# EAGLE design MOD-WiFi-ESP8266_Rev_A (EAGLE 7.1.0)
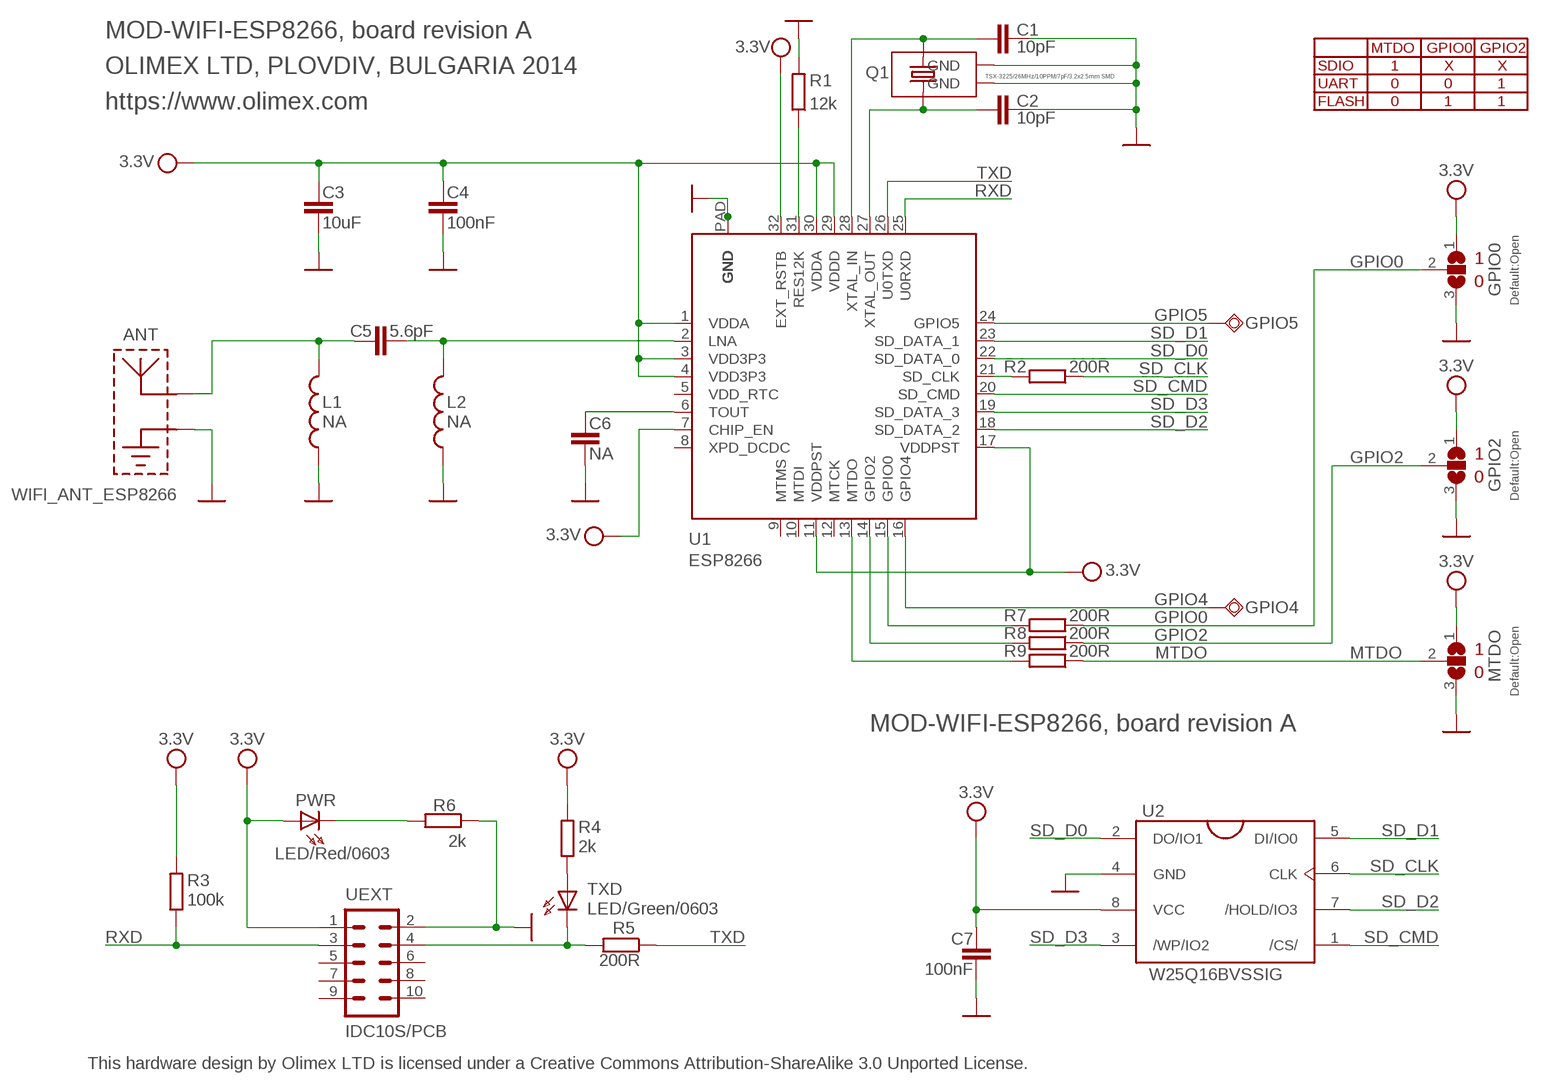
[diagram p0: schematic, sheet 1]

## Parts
ANT  WIFI_ANT_ESP8266  [ESP8266_ANT]
C1  10pF  C-EUC0402_TI  [C0402_TI]
C2  10pF  C-EUC0402_TI  [C0402_TI]
C3  10uF  C-EUC0603_DWS  [C0603_DWS]
C4  100nF  C-EUC0402_TI  [C0402_TI]
C5  5.6pF  C-EUC0402_TI  [C0402_TI]
C6  NA  C-EUC0402_TI  [C0402_TI]
C7  100nF  C-EUC0402_TI  [C0402_TI]
GPIO0  Default:Open  SJ2W4  [SJ_2_SMALLER]
GPIO2  Default:Open  SJ2W4  [SJ_2_SMALLER]
GPIO4  TESTPAD32/56  [TESTPAD32/56]
GPIO5  TESTPAD32/56  [TESTPAD32/56]
L1  NA  L-USL0402_TI  [L0402_TI]
L2  NA  L-USL0402_TI  [L0402_TI]
MTDO  Default:Open  SJ2W4  [SJ_2_SMALLER]
PWR  LED/Red/0603  LED0603DWS  [LED-0603]
Q1  TSX-3225/26MHz/10PPM/7pF/3.2x2.5mm SMD  SMALL_SMD_CRYSTAL_1  [NX3225SA]
R1  12k  R-EU_R0402_TI  [R0402_TI]
R2  200R  R-EU_R0402_TI  [R0402_TI]
R3  100k  R-EU_R0402_TI  [R0402_TI]
R4  2k  R-EU_R0402_TI  [R0402_TI]
R5  200R  R-EU_R0402_TI  [R0402_TI]
R6  2k  R-EU_R0402_TI  [R0402_TI]
R7  200R  R-EU_R0402_TI  [R0402_TI]
R8  200R  R-EU_R0402_TI  [R0402_TI]
R9  200R  R-EU_R0402_TI  [R0402_TI]
TXD  LED/Green/0603  LED0603DWS_L  [LED-0603_L]
U1  ESP8266  [QFN32_PAD]
U2  W25Q16BVSSIG  [SO8_ATMEL_FLASH]
UEXT  IDC10S/PCB  ML10SMD_1  [ML10L_PADS_FEMAIL]

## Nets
GND: ANT.GND C1.1 C2.1 C3.2 C4.2 C6.2 C7.2 GPIO0.3 GPIO2.3 L1.1 L2.1 MTDO.3 Q1.NC_1(GND) Q1.NC_2(GND) R1.2 R6.1 U1.P$1(GND) U1.P$2(GND) U1.P$3(GND) U1.P$4(GND) U1.P$5(GND) U1.P$6(GND) U1.P$7(GND) U1.P$8(GND) U1.P$9(GND) U1.PAD(GND) U2.4(GND) UEXT.2
GPIO0: GPIO0.2 R7.1
GPIO2: GPIO2.2 R8.1
GPIO4: GPIO4.P$1(PP) U1.16(GPIO4)
GPIO5: GPIO5.P$1(PP) U1.24(GPIO5)
MTDO: MTDO.2 R9.1
N$1: R5.2 TXD.C UEXT.4
N$2: R4.1 TXD.A
N$3: PWR.C R6.2
N$4: R7.2 U1.15(GPIO0)
N$5: R8.2 U1.14(GPIO2)
N$6: R9.2 U1.13(MTDO)
N$12: C5.2 L2.2 U1.2(LNA)
N$14: ANT.ANT C5.1 L1.2
N$18: C6.1 U1.6(TOUT)
N$21: C2.2 Q1.2 U1.27(XTAL_OUT)
N$22: R1.1 U1.31(RES12K)
N$23: C1.2 Q1.1 U1.28(XTAL_IN)
N$27: R2.2 U1.21(SD_CLK)
RXD: R3.1 U1.25(U0RXD) UEXT.3
SD_CLK: R2.1 U2.6(CLK)
SD_CMD: U1.20(SD_CMD) U2.1(/CS/)
SD_D0: U1.22(SD_DATA_0) U2.2(DO/IO1)
SD_D1: U1.23(SD_DATA_1) U2.5(DI/IO0)
SD_D2: U1.18(SD_DATA_2) U2.7(/HOLD/IO3)
SD_D3: U1.19(SD_DATA_3) U2.3(/WP/IO2)
TXD: R5.1 U1.26(U0TXD)
VCC: C3.1 C4.1 C7.1 GPIO0.1 GPIO2.1 MTDO.1 PWR.A R3.2 R4.2 U1.1(VDDA) U1.3(VDD3P3) U1.4(VDD3P3) U1.7(CHIP_EN) U1.11(VDDPST) U1.17(VDDPST) U1.29(VDDD) U1.30(VDDA) U1.32(EXT_RSTB) U2.8(VCC) UEXT.1 ; supply symbol labelled 3.3V
Unconnected: U1.5(VDD_RTC) U1.8(XPD_DCDC) U1.9(MTMS) U1.10(MTDI) U1.12(MTCK) UEXT.5 UEXT.6 UEXT.7 UEXT.8 UEXT.9 UEXT.10

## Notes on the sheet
- MOD-WIFI-ESP8266, board revision A
- MTDO | GPIO0 | GPIO2
- OLIMEX LTD, PLOVDIV, BULGARIA 2014 | SDIO | 1 | X | X
- UART | 0 | 0 | 1
- https://www.olimex.com | FLASH | 0 | 1 | 1
- 1
- 0
- 1
- 0
- 1
- 0
- MOD-WIFI-ESP8266, board revision A
- This hardware design by Olimex LTD is licensed under a Creative Commons Attribution-ShareAlike 3.0 Unported License.

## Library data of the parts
ANT = OLIMEX_ANT:WIFI_ANT_ESP8266
C1-C7 = rcl:C-EU: CAPACITOR, European symbol
GPIO0 GPIO2 MTDO = jumper:SJ2W: SMD solder JUMPER
GPIO4 GPIO5 = gogo:TESTPAD: drill 40mils, diameter 70mils
L1 L2 = rcl:L-US: INDUCTOR, American symbol
PWR TXD = DOUBLE-SIDE:LED
Q1 = OLIMEX_DISCRET:SMALL_SMD_CRYSTAL
R1-R9 = rcl:R-EU_: RESISTOR, European symbol
U1 = OLIMEX_IC:ESP8266
U2 = OLIMEX_IC:W25Q16BVSSIG
UEXT = con-harting-ml:ML10: HARTING

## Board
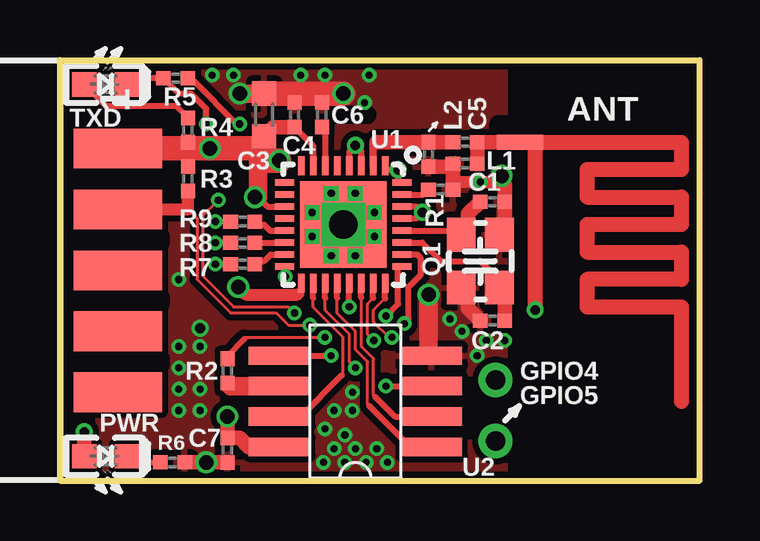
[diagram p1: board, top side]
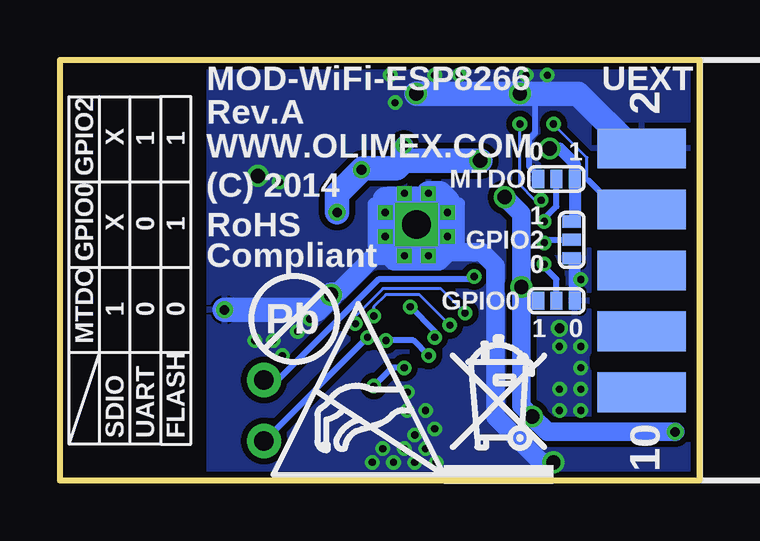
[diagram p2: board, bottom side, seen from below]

Size 26.67 x 17.53 mm. Coordinates in mm from the lower left corner, seen from the top.
Outline: 26.67,0 26.67,17.53 0,17.53 0,0 26.67,0
Copper layers (1+16): Top 0.035mm / dielectric 1.5mm / Bottom 0.035mm
Design rules "default": minimum track width 5mil, minimum drill 0.3mm, track to track 5mil, track to pad 5mil, pad to pad 5mil, via to via 5mil, smd to smd 1mil, copper to edge 5mil, drill to drill 8mil, minimum pad ring 6mil, minimum via ring 6mil, stop-mask expansion 2mil, vias tented up to drill 25mil, thermal gap 10mil
tRestrict: 6 lines
bRestrict: 7 lines

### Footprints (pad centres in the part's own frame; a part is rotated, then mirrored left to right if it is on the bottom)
ESP8266_ANT = smd 0.635 x 1.905: ANT -5.334,-3.302 | drill 0.4 pad 0.635: GND 1.651,-2.667
C0402_TI = smd 0.61 x 0.584: 1 -0.508,0; 2 0.508,0
C0603_DWS = smd 1.016 x 1.016: 1 -0.889,0; 2 0.889,0
SJ_2_SMALLER = smd 0.508 x 0.762: 1 -0.762,0; 2 0,0; 3 0.762,0
TESTPAD32/56 = drill 0.813 pad 1.422: P$1 0,0
L0402_TI = smd 0.61 x 0.584: 1 -0.508,0; 2 0.508,0
LED-0603 = smd 1.016 x 1.016: A 0.889,0; C -0.889,0
NX3225SA = smd 1.4 x 1.2: 1 -1.1,-0.8; 2 1.1,0.8; NC_1 1.1,-0.8; NC_2 -1.1,0.8
R0402_TI = smd 0.61 x 0.584: 1 -0.508,0; 2 0.508,0
LED-0603_L = smd 1.016 x 1.016: A 0.889,0; C -0.889,0
QFN32_PAD = smd 0.8 x 0.28: 1 -2.45,1.75; 2 -2.45,1.25; 3 -2.45,0.75; 4 -2.45,0.25; 5 -2.45,-0.25; 6 -2.45,-0.75; 7 -2.45,-1.25; 8 -2.45,-1.75; 17 2.45,-1.75; 18 2.45,-1.25; 19 2.45,-0.75; 20 2.45,-0.25; 21 2.45,0.25; 22 2.45,0.75; 23 2.45,1.25; 24 2.45,1.75 | smd 0.28 x 0.8: 9 -1.75,-2.45; 10 -1.25,-2.45; 11 -0.75,-2.45; 12 -0.25,-2.45; 13 0.25,-2.45; 14 0.75,-2.45; 15 1.25,-2.45; 16 1.75,-2.45; 25 1.75,2.45; 26 1.25,2.45; 27 0.75,2.45; 28 0.25,2.45; 29 -0.25,2.45; 30 -0.75,2.45; 31 -1.25,2.45; 32 -1.75,2.45 | drill 1.2 pad 1.422 square: P$1 0,0 | drill 0.3 pad 0.4 square: P$2 0.5,1.3; P$3 -0.5,1.3; P$4 -1.3,0.5; P$5 -1.3,-0.5; P$6 -0.5,-1.3; P$7 0.5,-1.3; P$8 1.3,-0.5; P$9 1.3,0.5 | smd 3.6 x 3.6: PAD 0,0
SO8_ATMEL_FLASH = smd 0.762 x 2.54: 1 -1.905,-3.175; 2 -0.635,-3.175; 3 0.635,-3.175; 4 1.905,-3.175; 5 1.905,3.175; 6 0.635,3.175; 7 -0.635,3.175; 8 -1.905,3.175
ML10L_PADS_FEMAIL = smd 1.651 x 3.683 bottom: 1 -5.08,-3.429; 3 -2.54,-3.429; 5 0,-3.429; 7 2.54,-3.429; 9 5.08,-3.429 | smd 1.651 x 3.683: 2 -5.08,-3.429; 4 -2.54,-3.429; 6 0,-3.429; 8 2.54,-3.429; 10 5.08,-3.429

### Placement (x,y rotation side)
ANT  22.48,8.76 270 top
C1  18.03,11.62 180 top
C2  18.03,6.67 0 top
C3  8.51,15.24 90 top
C4  9.78,15.24 90 top
C5  16.89,14.1 180 top
C6  10.92,15.24 90 top
C7  6.99,1.27 270 top
GPIO0  5.97,7.49 0 bottom
GPIO2  5.33,10.03 270 bottom
GPIO4  18.16,4.19 0 top
GPIO5  18.16,1.65 0 top
L1  16.89,13.21 0 top
L2  15.37,13.59 90 top
MTDO  5.97,12.57 180 bottom
PWR  1.91,1.02 180 top
Q1  17.53,9.14 270 top
R1  15.88,12.13 0 top
R2  6.99,4.57 90 top
R3  5.33,12.57 90 top
R4  5.33,14.61 270 top
R5  4.83,16.76 180 top
R6  4.7,0.76 180 top
R7  7.62,9.02 0 top
R8  7.62,9.91 0 top
R9  7.62,10.79 0 top
TXD  1.91,16.51 180 top
U1  11.81,10.67 270 top
U2  12.32,3.3 90 top
U$4  [ESD_SYMBOL]  17.78,0.25 0 bottom
U$6  [PB_SMALL]  16.89,6.73 180 bottom
U$7  [RECYCLE_BIN1/8]  10.67,-0.13 0 bottom
UEXT  -1.02,8.76 270 bottom

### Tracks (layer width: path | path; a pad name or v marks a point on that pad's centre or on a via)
GND  (via drill 0.3, 0.4, 0.6)
  Top 0.254: 17.02,8.04 Q1.NC_1
  Top 0.508: 16.38,12.45 18.41,12.45 v18.41,12.7
  Top 0.61: 16.38,13.08 L2.1 | R1.2 16.38,12.45 16.38,13.08 | 16.38,13.08 L1.1 | Q1.NC_2 18.54,10.46 C1.1 18.54,12.32 18.41,12.45 | C2.1 17.02,7.18 17.02,8.04 | R6.1 v6.1,0.76 C7.2 | 9.78,16.13 C4.2 | 10.92,16.13 C6.2
  Top 0.762: v15.37,7.75 15.37,5.21 U2.4 | v7.49,16.13 C3.2
  Top 1.016: C3.2 9.78,16.13 10.92,16.13 v11.81,16.13
  Bottom 0.254: MTDO.3 6.73,12.7 7.11,13.08 7.11,14.22 6.86,14.48 6.86,16.13
  Bottom 0.508: 13.11,11.72 12.95,11.87 | U1.P$5 11.31,11.87 | 12.31,11.87 U1.P$4 | 10.03,11.56 10.03,9.78 10.79,9.02 12.83,9.02 13.59,9.78 13.59,11.56 13.11,11.56 | GPIO0.3 5.21,9.27 GPIO2.3
  Bottom 0.762: v6.1,0.76 6.6,0.76 8.51,2.67 8.51,8.95 9.08,9.53 10.67,9.53 | 12.95,11.87 12.31,11.87 11.31,11.87 | 12.8,9.37 13.56,9.37 15.05,7.87 15.24,7.87 v15.37,7.75
  Bottom 1.016: UEXT.2 2.79,13.84 5.08,16.13 6.86,16.13 v7.49,16.13 v11.81,16.13 | 13.11,11.72 13.11,11.56 U1.P$3 U1.P$2 13.11,9.68 12.8,9.37 U1.P$9 U1.P$8 10.82,9.37 10.67,9.53 10.51,9.68 U1.P$7 10.51,10.67 | U1.P$5 10.82,11.97 10.51,11.65 U1.P$6 10.51,10.67 | 10.51,10.67 U1.P$1 | v15.37,7.75 16,7.11 ANT.GND
  other vias: 5.84,6.35 5.84,5.59 4.95,5.59 4.95,4.7 4.95,3.81 5.84,3.81 4.95,2.92 11.43,2.92 11.05,2.16 11.87,0.76 10.99,0.76 13.65,0.76 13.21,1.33 12.76,0.76 12.32,1.33 11.43,1.33 11.87,1.91 12.19,2.92 12.19,3.68 16.26,6.73 16.76,6.22 12.7,15.75 17.53,12.45 4.95,8.38 5.84,2.92 12.89,16.89 17.4,5.21 18.54,5.84 17.78,5.84 10.03,16.89 11.05,16.89 7.24,16.89 6.35,16.89
  pour Top (isolate 0.254): -2.54,-2.54 -2.54,20.07 29.21,20.07 29.21,-2.54
  pour Bottom (isolate 0.254): -5.08,-5.08 -5.08,22.61 31.88,22.61 31.88,-5.08
GPIO0  (via drill 0.3)
  Top 0.254: v6.48,9.02 R7.1
  Bottom 0.254: v6.48,9.02 6.48,8.89 5.97,8.38 GPIO0.2
GPIO2  (via drill 0.3)
  Top 0.254: R8.1 v6.48,9.91
  Bottom 0.254: v6.48,9.91 6.35,10.03 GPIO2.2
GPIO4  (via drill 0.3)
  Top 0.254: U1.16 9.4,8.92 v9.4,8.51
  Bottom 0.254: v9.4,8.51 9.53,8.38 13.4,8.38 17.59,4.19 GPIO4.P$1
GPIO5  (via drill 0.3)
  Top 0.127: 13.56,7.59 13.08,7.11 13.08,6.6 13.72,5.97 v13.84,5.97
  Top 0.254: 13.56,7.59 U1.24
  Bottom 0.254: GPIO5.P$1 v13.84,5.97
MTDO  (via drill 0.3)
  Top 0.254: R9.1 v6.48,10.79
  Bottom 0.254: v6.48,10.79 6.48,10.92 5.97,11.43 MTDO.2
N$1  (via drill 0.3)
  Top 0.254: TXD.C 3.05,16.76 R5.2 4.95,16.13 5.46,16.13 6.1,15.49 v6.1,14.86
  Bottom 0.127: UEXT.4 3.43,11.3 | 4.64,12.51 4.7,12.57 4.7,13.46 v6.1,14.86
  Bottom 0.254: 3.43,11.3 4.64,12.51
N$2
  Top 0.254: TXD.A 1.91,15.62 4.83,15.62 R4.1
N$3
  Top 0.254: PWR.C 3.05,0.76 R6.2
N$4
  Top 0.254: R7.2 8.26,9.14 8.51,9.14 8.78,9.42 U1.15
N$5
  Top 0.254: R8.2 U1.14
N$6
  Top 0.254: R9.2 8.26,10.67 8.51,10.67 8.76,10.42 U1.13
N$12
  Top 0.305: U1.2 13.06,13.95 13.21,14.1
  Top 0.61: C5.2 L2.2 13.21,14.1
N$14
  Top 0.61: L1.2 C5.1 ANT.ANT
N$18
  Top 0.254: C6.1 11.06,14.59 U1.6
N$21
  Top 0.254: U1.27 15.1,9.92 15.88,9.14 17.53,9.14 18.33,8.34 Q1.2
  Top 0.61: C2.2 18.54,7.83 Q1.2
N$22
  Top 0.254: U1.31 15.16,11.92 R1.1
N$23
  Top 0.254: 17.02,10.24 Q1.1 | U1.28 17.02,10.42
  Top 0.61: 17.02,10.24 17.02,10.42 17.02,11.11 C1.2
N$27  (via drill 0.3)
  Top 0.127: v12.06,7.24 | R2.2 6.99,5.21 | 7.68,5.91 7.75,5.97 v11.05,5.97
  Top 0.254: v12.06,7.24 U1.21 | 6.99,5.21 7.68,5.91
  Bottom 0.254: v11.05,5.97 11.05,6.22 v12.06,7.24
RXD  (via drill 0.3)
  Top 0.127: 5.33,11.3 5.71,10.92 5.71,8.38 7.11,6.99 9.02,6.99 9.53,6.48 v10.41,6.48
  Top 0.254: v13.59,6.86 14.1,7.37 14.1,8.38 14.1,8.92 U1.25
  Top 0.508: UEXT.3 5.33,11.3 R3.1
  Bottom 0.127: v10.41,6.48 11.68,7.75 13.08,7.75 13.59,7.24 v13.59,6.86
SD_CLK
  Top 0.61: R2.1 7.11,3.94
  Top 0.762: 7.11,3.94 U2.6
SD_CMD
  Top 0.127: 12.89,3.11 12.83,3.17 12.83,4.95 12.32,5.46 12.32,6.22 11.56,6.98 11.56,7.62
  Top 0.254: 11.56,7.62 U1.20 | U2.1 14.61,1.4 12.89,3.11
SD_D0
  Top 0.127: 12.56,7.63 12.57,7.62 12.57,5.59 13.08,5.08 13.08,3.56 13.14,3.49
  Top 0.254: 12.56,7.63 U1.22 | 13.14,3.49 13.97,2.67 U2.2
SD_D1  (via drill 0.3)
  Top 0.127: v13.08,5.84 12.83,6.1 12.83,7.37 13.06,7.6
  Top 0.254: 13.06,7.6 U1.23 | U2.5 v11.3,5.21
  Bottom 0.254: v11.3,5.21 11.94,5.84 v13.08,5.84
SD_D2
  Top 0.127: 11.75,4.38 11.81,4.45 11.81,5.97 10.56,7.22 10.56,7.6 | U2.7 10.03,2.67
  Top 0.254: 10.56,7.6 U1.18 | 10.03,2.67 11.75,4.38
SD_D3  (via drill 0.3)
  Top 0.127: v12.32,4.7 12.06,4.95 12.06,6.1 11.06,7.1 11.06,7.61
  Top 0.254: 11.06,7.61 U1.19 | v13.59,3.94 U2.3
  Bottom 0.254: v12.32,4.7 12.83,4.7 v13.59,3.94
TXD  (via drill 0.3)
  Top 0.127: v6.6,11.68 5.97,11.05 5.97,8.51 7.24,7.24 9.53,7.24 v9.78,6.99
  Top 0.254: U1.26 14.9,9.42 15.05,9.27 15.05,8.57 14.54,8.06 14.54,6.73 v14.35,6.54 | v7.49,14.86 7.37,14.86 5.59,16.64 5.21,16.64 R5.1
  Bottom 0.127: v6.6,11.68 6.86,11.68 7.49,12.32 v7.49,14.86 | v14.35,6.54 14.35,6.86 13.21,8 10.79,8 v9.78,6.99
VCC  (via drill 0.4, 0.6)
  Top 0.254: C4.1 10.56,13.95 U1.7 | U1.4 12.06,13.71 v12.32,13.97 12.56,13.73 U1.3 | U1.1 13.56,12.95 v14.1,12.95 14.1,12.42 U1.32 | U1.30 14.87,11.42 v15.11,11.18 14.86,10.92 U1.29 | 9.91,7.75 10.06,7.75 U1.17 | 8.26,11.81 8.65,11.42 U1.11
  Top 0.508: v7.43,8.06 7.75,7.75 9.91,7.75
  Top 0.61: PWR.A v1.02,2.03 | v6.99,2.67 C7.1 7.49,1.78 7.87,1.4 U2.8 | C3.1 8.89,14.73 C4.1 | R4.2 5.33,13.84 R3.2
  Top 0.762: v8.13,11.81 8.26,11.81 8.26,13.34 v9.14,13.34
  Top 1.016: 8.51,13.84 C3.1 | v9.14,13.34 8.51,13.34 8.51,13.84 | 8.51,13.84 v6.25,13.84 5.33,13.84 UEXT.1
  Bottom 0.508: 6.86,7.49 GPIO0.1 | GPIO2.1 5.21,10.79 MTDO.1 5.21,13.21 5.84,13.84 v6.25,13.84
  Bottom 0.762: v1.02,2.03 6.35,2.03 v6.99,2.67 7.43,3.11 7.43,7.49 | 7.43,7.49 6.86,7.49 | 7.43,7.49 v7.43,8.06 7.43,11.11 v8.13,11.81 | 12.32,13.34 v12.32,13.97
  Bottom 1.016: v9.14,13.34 12.32,13.34 12.64,13.02 14.03,13.02 v14.1,12.95 15.11,11.94 v15.11,11.18

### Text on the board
bPlace: 1 | 1 | X | GPIO2 | 1 | 0 | X | GPIO0 | 0 | 0 | 1 | MTDO | FLASH | UART | SDIO
bNames: MOD-WiFi-ESP8266 | Rev.A | 1 | 0 | WWW.OLIMEX.COM | (C) 2014 | 1 | RoHS | 0 | Compliant | 0 | 1 | 10
201bmp: C:/YASSEN_ON_C-YASSEN-REBORN/TASKS/MOD-nRF8001===P/Nordic_NRF8001/nRF8001-Gerber Files/with DCDC/\!PICLIST-0909+++.BMP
